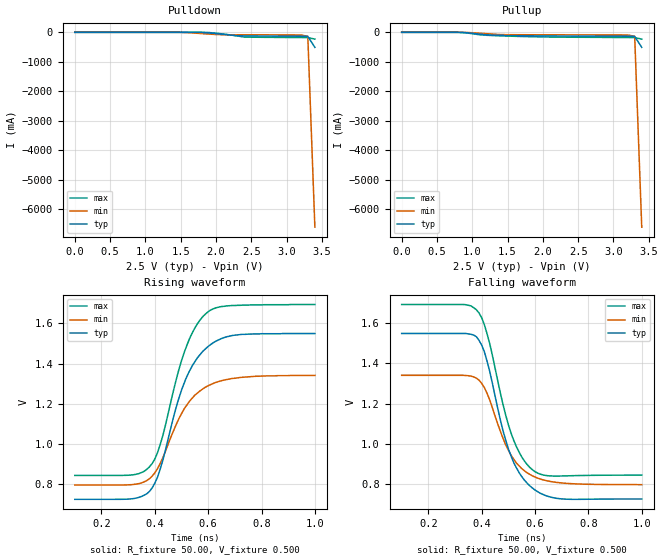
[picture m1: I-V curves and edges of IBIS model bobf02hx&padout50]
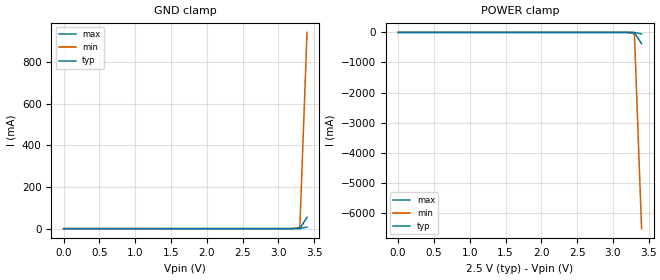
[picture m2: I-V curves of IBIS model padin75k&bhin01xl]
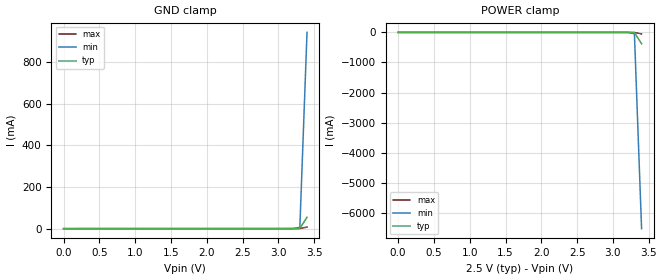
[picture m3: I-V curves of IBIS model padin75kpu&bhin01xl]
|   This file is an IBIS representation of the   |
|   Integrated Device Technology, Inc.   |
|   MC100ES6014   |
|   Dual 2:1 Differential Multiplexer   |
[IBIS Ver]   3.2
[File name]   mc100es6014_2v5.ibs
[File Rev]   0.01
[Date]   29 November 2007 | Last modified
|   29 November 2007 | Generated
[Source]   Originated at Integrated Device Technology, Inc.
[Disclaimer]
   (C) Copyright Integrated Device Technology, Inc. 2005
   All rights reserved
   IDT hereby grants the user of this IBIS model a non-exclusive,
   nontransferable license to use this IBIS model under the following terms.
   Before using this IBIS model, the user should read this license.
   If the user does not accept these terms,  the IBIS model should be
   returned to IDT within 30 days.
   The user is granted this license only to use the IBIS model and
   is not granted rights to sell, load, rent, lease or license the IBIS
   model in whole or in part, or in modified form to anyone other than
   user. User may modify the IBIS model to suit its specific
   applications but rights to derivative works and such modifications
   shall belong to IDT.
   This IBIS model is provided on an "AS IS" basis and IDT makes
   absolutely no warranty with respect to the information contained
   herein. IDT DISCLAIMS AND CUSTOMER WAIVES ALL WARRANTIES, EXPRESS
   OR IMPLIED, INCLUDING WARRANTIES OF MERCHANTABILITY OR FITNESS FOR
   A PARTICULAR PURPOSE. The entire risk as to quality and performance
   is with the Customer. ACCORDINGLY, IN NO EVENT SHALL THE COMPANY BE
   LIABLE FOR ANY DAMAGES, WHETHER IN CONTRACT OR TORT,INCLUDING ANY
   LOST PROFITS OR OTHER INCIDENTAL, CONSEQUENTIAL, EXEMPLARY, OR
   PUNITIVE DAMAGES ARISING OUT OF THE USE OR APPLICATION OF THE IBIS
   model provided in this package. Further, IDT reserves the right to
   make changes without notice to any product herein to improve
   reliability, function, or design. IDT does not convey any license
   under patent rights or any other intellectual property rights,
   including those of third parties.
   IDT is not obligated to provide maintenance or support
   for the licensed IBIS model.
[Copyright]   Copyright 2002 by Integrated Device Technology, Inc.
[Component]   20ld_TSSOP
[Manufacturer]   Integrated Device Technology, Inc.
[Package]
   |TSSOP20
   |   typ   min   max
   R_pkg   220.4m   212.5m   238m
   L_pkg   1.841n   1.708n   1.974n
   C_pkg   0.316p   0.2907p   0.33p
[Pin]   signal_name   model_name
   1   Q0   bobf02hx&padout50
   2   nQ0   bobf02hx&padout50
   3   Q1   bobf02hx&padout50
   4   nQ1   bobf02hx&padout50
   5   Q2   bobf02hx&padout50
   6   nQ2   bobf02hx&padout50
   7   Q3   bobf02hx&padout50
   8   nQ3   bobf02hx&padout50
   9   Q4   bobf02hx&padout50
   10   nQ4   bobf02hx&padout50
   11   VEE   GND
   12   COM_SEL   padin75k&bhin01xl
   13   CLK0   padin75k&bhin01xl
   14   nCLK0   padin75kpu&bhin01xl
|   15   VBB   Bias
   16   CLK1   padin75k&bhin01xl
   17   nCLK1   padin75kpu&bhin01xl
   18   VCC   POWER
   19   nEN   padin75k&bhin01xl
   20   VCC   POWER
[Diff Pin]   inv_pin  vdiff tdelay_typ tdelay_min  tdelay_max
   13   14   0.0   0   0   0
   16   17   0.0   0   0   0
   1   2   NA   0   0   0
   3   4   NA   0   0   0
   5   6   NA   0   0   0
   7   8   NA   0   0   0
   9   10   NA   0   0   0
| Models and submodels in the file (3): bobf02hx&padout50 (Output_ECL), padin75k&bhin01xl (Input), padin75kpu&bhin01xl (Input)
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[Model]   bobf02hx&padout50
   Model_type  Output_ECL
   Polarity   Non-Inverting
   C_comp   1.0p   0.5p   1.5p
   Vmeas =   1.2
   Rref =   50.0
   Cref =   0.0
   Vref =   0.5
[Temperature range]   25.0   -40.0   85.0
[Voltage Range]   2.500   2.375   2.652
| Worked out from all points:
|   rising waveform, R_fixture 50.00, V_fixture 0.500: 20-80 % time 115ps typ, 122ps min, 106ps max; typ from 0.726 V to 1.55 V
|   falling waveform, R_fixture 50.00, V_fixture 0.500: 20-80 % time 101ps typ, 104ps min, 96.1ps max; typ from 1.55 V to 0.726 V
   |  Voltage   I(typ)   I(min)   I(max)
[Pullup]
0V        232.2fA    86.23fA    9.071pA
800mV     -579.4uA   -33.06uA   -1.212mA
1.2V      -84.35mA   -45.91mA   -99.55mA
1.8V      -119.6mA   -82.73mA   -147.7mA
3.2V      -132.1mA   -89.62mA   -176mA
3.3V      -140.4mA   -135mA     -178.8mA
3.4V      -510mA     -6.612A    -230mA
[Pulldown]|
0V        235.3fA    87.5fA     9.078pA
1.5V      -95.86nA   -1.148mA   -44.71nA
1.8V      -4.189mA   -42.87mA   -458.5uA
2V        -44.11mA   -74.17mA   -28.01mA
2.4V      -123.4mA   -84.05mA   -161.7mA
3.2V      -132.1mA   -89.64mA   -176.1mA
3.3V      -140.4mA   -135.1mA   -178.9mA
3.4V      -510mA     -6.612A    -230.1mA
[Ramp]
   |   typ   min   max
   dV/dt_r   0.70V/0.2ns   0.60V/0.20ns   0.84V/0.20ns
   dV/dt_f   0.70V/0.2ns   0.60V/0.20ns   0.84V/0.20ns
   R_load =   50.0000
[Rising Waveform]
   R_fixture =   50.00
   V_fixture =   0.500
   V_fixture_min =  0.375
   V_fixture_max =  0.625
| time(s)   voltage(typ)   voltage(min)   voltage(max)
100ps     726.3mV    797.4mV    844.9mV
320ps     730mV      800.1mV    848.2mV
390ps     783.1mV    841.3mV    903.6mV
430ps     920.1mV    932.6mV    1.042V
480ps     1.183V     1.097V     1.319V
520ps     1.336V     1.194V     1.49V
560ps     1.429V     1.254V     1.598V
600ps     1.485V     1.29V      1.657V
700ps     1.541V     1.327V     1.688V
1ns       1.549V     1.341V     1.693V
[Falling Waveform]
   R_fixture =   50.00
   V_fixture =   0.500
   V_fixture_min =  0.375
   V_fixture_max =  0.625
|   time(s)   voltage(typ)   voltage(min)   voltage(max)
100ps     1.549V     1.341V     1.693V
340ps     1.549V     1.34V      1.692V
390ps     1.515V     1.317V     1.651V
430ps     1.361V     1.219V     1.499V
470ps     1.119V     1.063V     1.253V
500ps     975.4mV    969.3mV    1.096V
540ps     857.5mV    891.1mV    959.6mV
590ps     780.8mV    841.3mV    871.5mV
700ps     726.6mV    805.9mV    840.5mV
1ns       726.3mV    797.5mV    844.8mV
|..............................................................................|
| .  .  .  .  .  .  .  .  .  .  .  .  .  .  .  .  .  .  .  .  .  .  .  .  .  . |
|..............................................................................|
[Model]   padin75k&bhin01xl
   Model_type   Input
   Polarity   Non-Inverting
   Vinl =   0.6V
   Vinh =   0.9V
   C_comp   1.0p   0.5p   1.5p
[Temperature range]   25.0   -40.0   85.0
[Voltage Range]   2.500   2.375   2.625
   |  Voltage   I(typ)   I(min)   I(max)
[GND_clamp]
0V        -52.9uA    -90.14uA   -34.56uA
3.2V      65.18uA    83.59uA    56.78uA
3.3V      1.153mA    6.537mA    342.1uA
3.4V      54.43mA    942.8mA    7.594mA
[POWER_clamp]
0V        33.24uA    28.8uA     37.09uA
3.2V      -281.2uA   -494.7uA   -162.7uA
3.3V      -7.911mA   -45.25mA   -2.214mA
3.4V      -376.6mA   -6.521A    -52.54mA
|..............................................................................|
| .  .  .  .  .  .  .  .  .  .  .  .  .  .  .  .  .  .  .  .  .  .  .  .  .  . |
|..............................................................................|
[Model]   padin75kpu&bhin01xl
   Model_type   Input
   Polarity   Non-Inverting
   Vinl =   0.6V
   Vinh =   0.9V
   C_comp   1.0p   0.5p   1.5p
[Temperature range]   25.0   -40.0   85.0
[Voltage Range]   2.500   2.375   2.625
   |  Voltage   I(typ)   I(min)   I(max)
[GND_clamp]
0V        -86.14uA   -119uA     -71.65uA
3.2V      74.48uA    93.59uA    64.91uA
3.3V      1.164mA    6.549mA    351.6uA
3.4V      54.44mA    942.8mA    7.605mA
[POWER_clamp]
0V        33.24uA    28.8uA     37.09uA
3.2V      -323.7uA   -533.5uA   -207.9uA
3.3V      -7.955mA   -45.29mA   -2.26mA
3.4V      -376.6mA   -6.521A    -52.58mA
